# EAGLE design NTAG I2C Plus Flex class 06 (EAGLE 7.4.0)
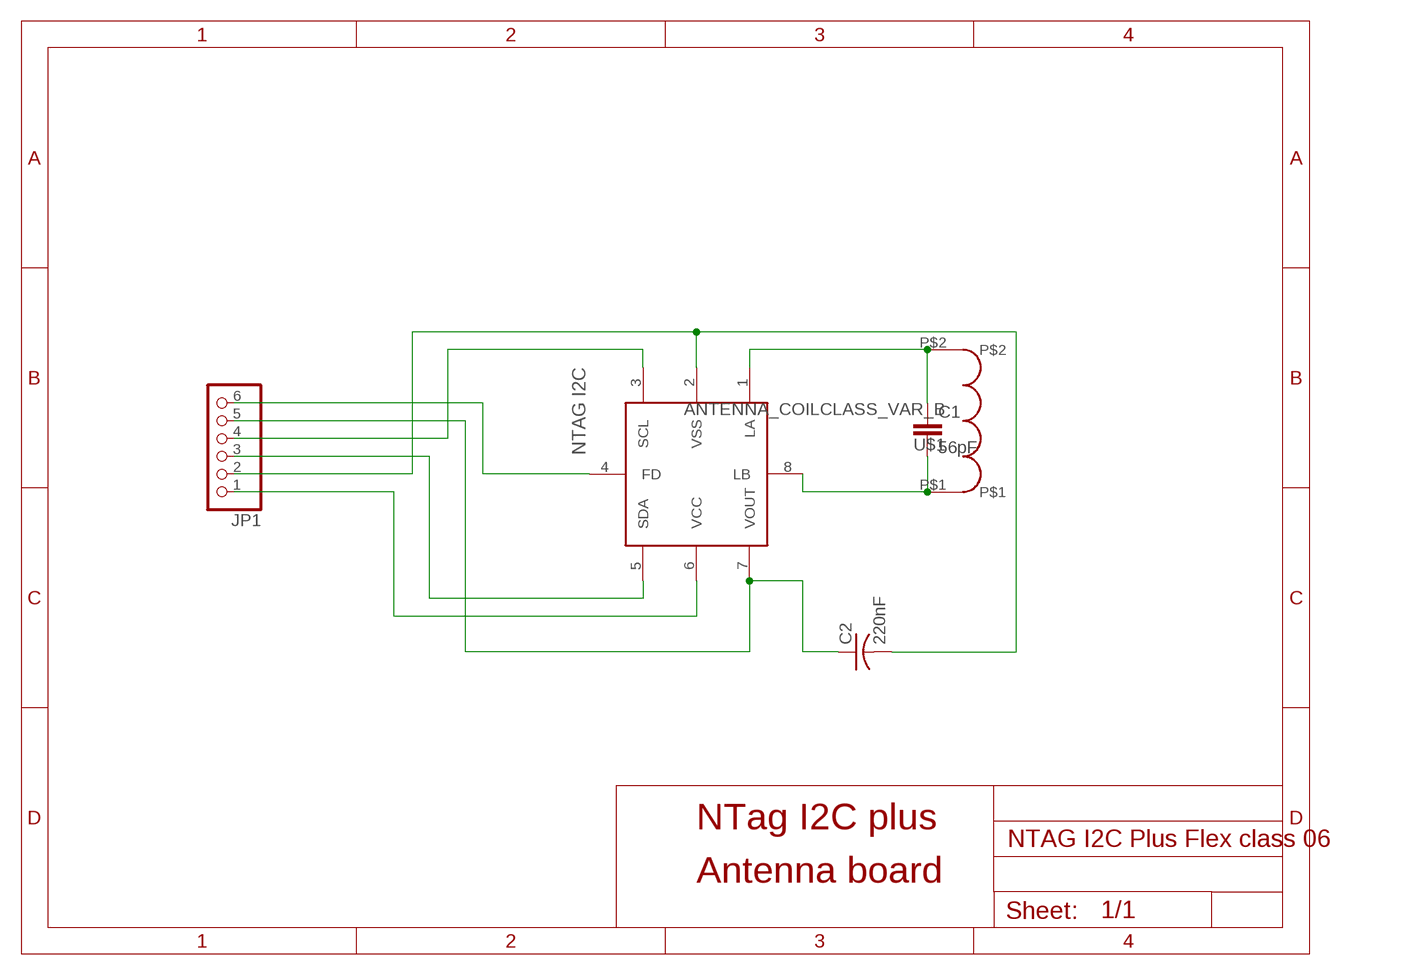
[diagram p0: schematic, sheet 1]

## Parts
C1  56pF  C-EUC0603  [C0603]
C2  220nF  C-USC0805  [C0805]
JP1  PINHD-1X6/90  [1X06/90]
NTAGUI  NTAG_I2C  [XQFN8]
U$1  ANTENNA_COILCLASS_VAR_B  [L_PICC_50PF_CLASS6_B]

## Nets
+VCC: JP1.1 NTAGUI.6(VCC)
FD: JP1.6 NTAGUI.4(FD)
N$1: C1.1 NTAGUI.1(LA) U$1.P$2
N$2: C1.2 NTAGUI.8(LB) U$1.P$1
N$8: JP1.4 NTAGUI.3(SCL)
SDA: JP1.3 NTAGUI.5(SDA)
VOUT: C2.1 JP1.5 NTAGUI.7(VOUT)
VSS: C2.2 JP1.2 NTAGUI.2(VSS)

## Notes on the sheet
- NTag I2C plus
- Antenna board

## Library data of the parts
C1 = rcl:C-EU: CAPACITOR, European symbol
C2 = rcl:C-US: CAPACITOR, American symbol
JP1 = pinhead (2):PINHD-1X6: PIN HEADER
NTAGUI = NTAG I2C:NTAG_I2C
U$1 = NXP_PICC_Antennas:ANTENNA_COIL: Antenna coils designs for Class 4, Class 5 and Class 6

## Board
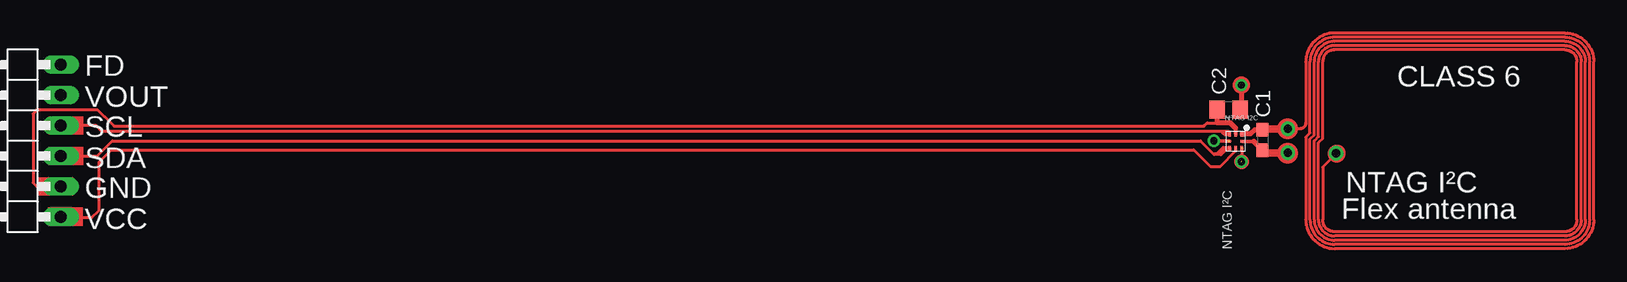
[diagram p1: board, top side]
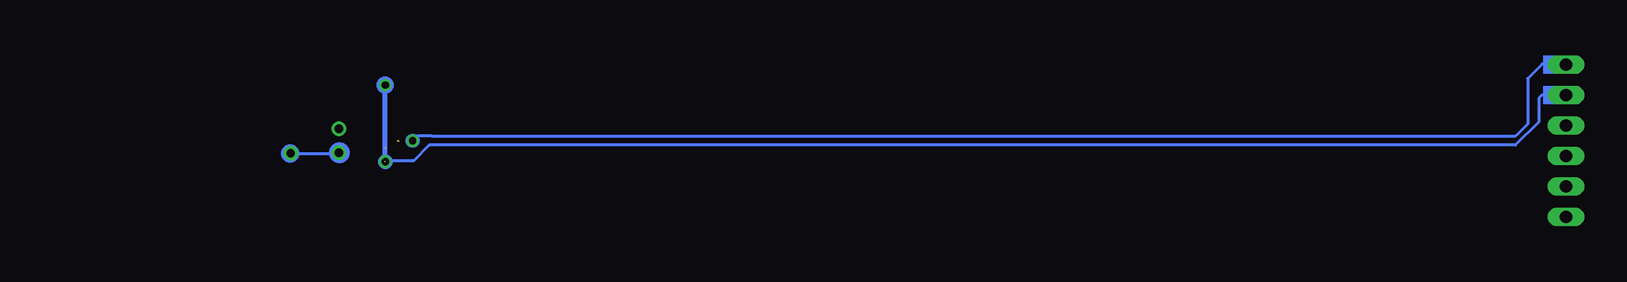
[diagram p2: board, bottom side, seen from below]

No outline drawn. Coordinates in mm, seen from the top.
Copper layers (1*16): Top 0.035mm / dielectric 1.5mm / Bottom 0.035mm
Design rules "default": minimum track width 10mil, minimum drill 24mil, track to track 8mil, track to pad 8mil, pad to pad 8mil, via to via 8mil, smd to smd 8mil, copper to edge 40mil, drill to drill 8mil, minimum pad ring 10mil, minimum via ring 8mil, stop-mask expansion 4mil, vias tented up to drill 0mil, thermal gap 10mil

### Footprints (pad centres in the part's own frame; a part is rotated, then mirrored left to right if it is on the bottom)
C0603 = smd 1.1 x 1: 1 -0.85,0; 2 0.85,0
C0805 = smd 1.3 x 1.5: 1 -0.95,0; 2 0.95,0
1X06/90 = drill 1.016 long: 1 -6.35,-3.81; 2 -3.81,-3.81; 3 -1.27,-3.81; 4 1.27,-3.81; 5 3.81,-3.81; 6 6.35,-3.81
XQFN8 = smd 0.4 x 0.32: 1 -0.6,0.55 | smd 0.4 x 0.22: 2 -0.6,0; 3 -0.6,-0.5; 5 0.6,-0.5; 6 0.6,0; 7 0.6,0.5 | smd 0.22 x 0.4: 4 0,-0.6; 8 0,0.6
L_PICC_50PF_CLASS6_B = drill 0.7: P$1 13.5,1; P$2 13.5,-1; P$3 9.48,1.05

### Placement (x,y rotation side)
C1  111.19,14.56 270 top
C2  108.36,17.09 180 top
JP1  7.2,14.5 90 top
NTAGUI  108.94,14.46 270 top
U$1  126.8,14.5 180 top

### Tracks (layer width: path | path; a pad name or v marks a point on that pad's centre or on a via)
+VCC
  Top 0.254: JP1.1 11.06,8.1 13.6,8.1 14.2,8.7 14.2,12.72 15.23,13.75 105.46,13.75 106.89,12.33 107.64,12.33 108.94,13.63 108.94,13.64 NTAGUI.6
FD  (via drill 0.6)  (3 unrouted)
  Top 0.254: v107.15,14.5 108.45,14.5 108.45,14.45 107.2,14.45 v107.15,14.5 | v107.15,14.5 v107.14,14.5
  Bottom 0.254: JP1.6 11.06,20.9 13,20.9 14.2,19.7 14.2,15.9 15.2,14.9 105.55,14.91 106.74,14.91 v107.14,14.5
N$1
  Top 0.254: 111.28,15.5 arc90 C1.1
  Top 0.406: C1.1 110.53,15.41 110.19,15.07 NTAGUI.1
  Top 0.61: U$1.P$2 111.19,15.5 C1.1
N$2
  Top 0.254: NTAGUI.8 110.44,14.46 | 109.45,14.45 110.45,14.45
  Top 0.406: C1.2 110.45,14.45 110.44,14.46
  Top 0.61: U$1.P$1 111.19,13.5 C1.2
N$3
  Top 0.254: 108.95,15.65 108.95,15.6 108.95,14.95
N$7
  Top 0.254: 108.35,13.8 108.2,13.8 108.15,13.75 | 108.15,13.75 107.75,13.35 107.75,13.8 107.9,13.95 108.45,13.95 108.45,13.75 108.15,13.75
N$8
  Top 0.254: 107.6,15.3 108.35,15.3 108.4,15.25 108.4,15 108.05,15 107.95,15.1 | JP1.4 13.95,15.77 14.44,15.28 107.79,15.28 107.79,15.26 107.9,15.15 107.95,15.1 | 108.01,15.06 NTAGUI.3 108.4,15.1 107.95,15.1
N$9
  Top 0.254: 108.95,13.65 108.95,13.7 108.95,13.95
N$10
  Top 0.254: 107.8,13.8 107.75,13.8 107.35,13.4 107.45,13.4 107.55,13.5
N$11
  Top 0.254: 107.55,13.4 107.2,13.4
SDA
  Top 0.254: JP1.3 13.28,13.23 13.29,13.22 14.05,13.22 15.31,14.49 106.01,14.49 107.15,13.35 107.71,13.35 107.85,13.49 107.85,13.65 | 107.85,13.86 107.85,13.65 | NTAGUI.5 108.06,13.86 107.85,13.65
VOUT  (via drill 0.6)  (2 unrouted)
  Top 0.254: 109.45,13.3 109.45,12.8 | 109.45,13.95 109.45,13.3 | 109.45,13.3 109.5,13.25
  Top 0.406: v109.44,12.75 v109.43,12.75 | v109.43,19.15 109.43,17.09 C2.1
  Bottom 0.254: JP1.5 13.01,18.31 13.27,18.05 13.27,16.08 15.22,14.13 105.76,14.13 107.06,12.83 109.35,12.83 v109.43,12.75
  Bottom 0.406: v109.43,12.75 v109.43,19.15
VSS
  Top 0.254: JP1.2 9.01,10.69 8.7,11 8.7,16.75 9,17.05 14.1,17.05 14.67,16.48 14.7,16.48 15.46,15.72 106.32,15.72 106.6,16 107.4,16 | NTAGUI.2 108.94,15.57
  Top 0.406: C2.2 107.41,16.01 107.4,16 108.51,16 108.94,15.57
(copper drawn outside any net)
  shapes: Bottom area x2, Bottom circle x15, Top area x4, Top circle x24

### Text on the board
tNames: FD | CLASS 6 | VOUT | SCL | SDA | GND | NTAG I²C | Flex antenna | VCC | NTAG I²C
